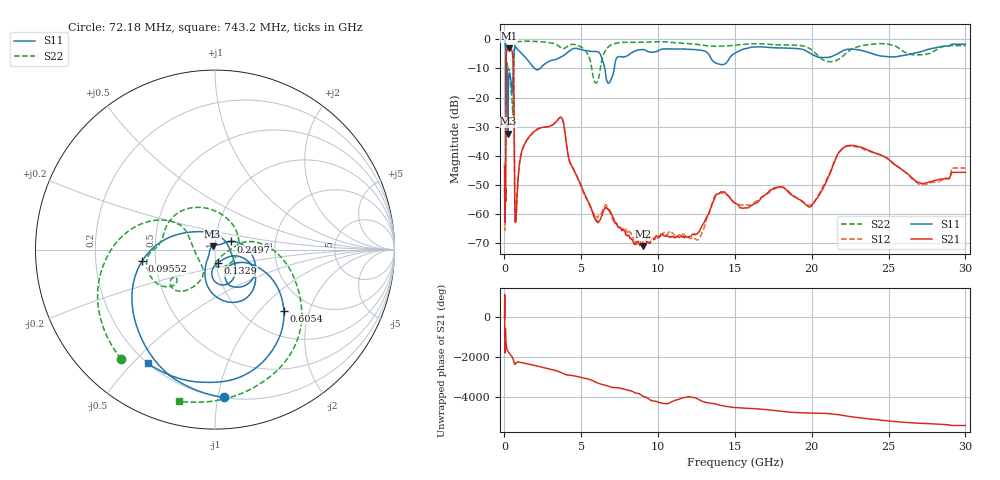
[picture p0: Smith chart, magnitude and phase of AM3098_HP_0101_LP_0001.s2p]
! Date/Time: Thu, Feb 28, 2019 8:36 AM
! Network Analyzer: Agilent Technologies E8364B Rev: A.07.50.67
! Sweep from 0.010 to 30.000 GHz, 1601 Points, Sweep Type: LOG
! Power Supply: 5.023 V, 0.002 A
# Hz S DB R 50
!freq MagS11 AngS11 MagS21 AngS21 MagS12 AngS12 MagS22 AngS22
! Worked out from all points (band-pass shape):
!   1601 points, 10 MHz to 30 GHz, reference 50 ohm
!   highest |S21| = -3.01 dB at 273.2 MHz (marker M1); lowest = -71.2 dB at 9.027 GHz (marker M2)
!   |S21| within 3 dB of the highest: 113.4 MHz to 546.4 MHz (432.9 MHz wide, 131 % of centre)
!   lowest |S11| = -32.5 dB at 230.5 MHz (marker M3), VSWR 1.05, Z = 48.7 + j1.91 ohm
!   |S11| at or under -10 dB: 176.1 MHz to 571.3 MHz (395.2 MHz wide, 106 % of centre); 1.965 GHz to 2.33 GHz (364.8 MHz wide, 17 % of centre); 6.532 GHz to 7.148 GHz (615.3 MHz wide, 9 % of centre)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
!   |S22| runs from -25.9 to -0.5 dB; largest |S21 - S12| = 0.012
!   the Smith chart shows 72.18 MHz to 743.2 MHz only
!   S11 on the Smith chart (normalised r, x): 72.18 MHz: 0.20, -1.04; 95.52 MHz: 0.42, -0.06; 132.9 MHz: 1.02, -0.15; 249.7 MHz: 1.19, +0.11; 605.4 MHz: 1.48, -1.38; 743.2 MHz: 0.20, -0.55
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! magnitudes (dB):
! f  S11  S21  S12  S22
! 10 MHz  -0.4  -43.7  -42.8  -0.5
! 38.04 MHz  -0.5  -59.9  -57.9  -0.8
! 72.18 MHz  -1.7  -54.7  -53.5  -1.9
! 95.52 MHz  -7.7  -21.5  -21.5  -9.3
! 132.9 MHz  -22.3  -4.2  -4.2  -11.1
! 144.7 MHz  -16.8  -3.8  -3.7  -11.0
! 186.8 MHz  -11.2  -3.5  -3.5  -8.2
! 230.5 MHz  -32.5  -3.1  -3.1  -10.0
! 249.7 MHz  -20.1  -3.1  -3.0  -10.3
! 273.2 MHz  -14.5  -3.0  -3.0  -10.5
! 550.5 MHz  -13.5  -6.3  -6.2  -25.9
! 605.4 MHz  -5.8  -15.5  -15.5  -11.4
! 679.2 MHz  -2.6  -58.4  -58.8  -2.2
! 743.2 MHz  -2.7  -61.8  -60.8  -1.2
! 2.084 GHz  -10.4  -31.1  -31.1  -0.7
! 3.704 GHz  -6.0  -26.9  -26.8  -2.9
! 5.959 GHz  -4.2  -62.2  -60.9  -15.0
! 7.926 GHz  -5.8  -67.4  -65.6  -1.0
! 9.027 GHz  -3.5  -71.2  -69.7  -1.0
! 19.8 GHz  -4.5  -57.7  -57.1  -2.9
! 22.67 GHz  -3.4  -36.5  -36.8  -3.2
! 30 GHz  -1.7  -45.8  -44.3  -2.1
